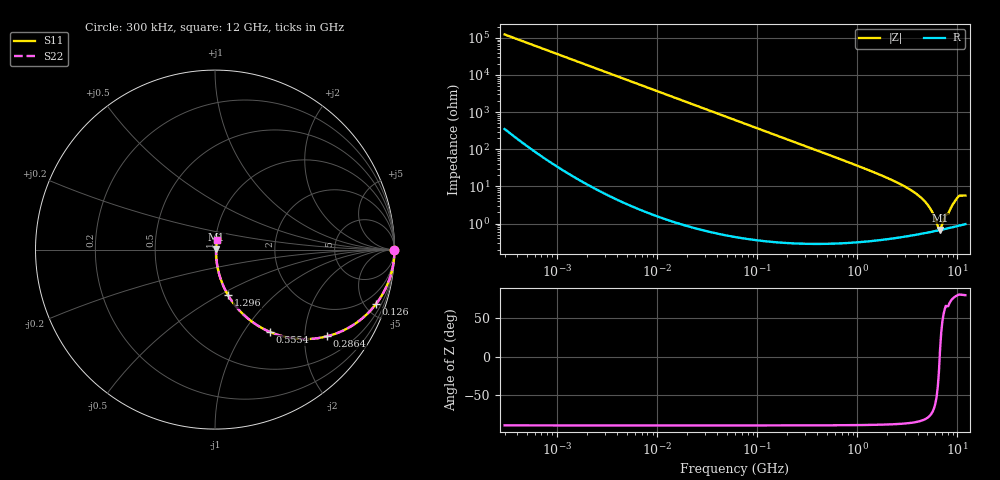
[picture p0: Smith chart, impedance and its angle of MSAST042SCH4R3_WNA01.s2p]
! MSAST042SCH4R3_WNA01  S-PARAMETER MODEL  ( General Type )
! Model Generated by TAIYO YUDEN Corporation (http://www.ty-top.com)
! Version 1.0
! TAIYO YUDEN Control No. 150820
! Copyright(c) 2015 TAIYO YUDEN CO.,LTD. All Rights Reserved.
! Product Description (link to TY-COMPAS)
! https://ds.yuden.co.jp/TYCOMPAS/or/detail?pn=MSAST042SCH4R3BWNA01&u=M
! Products Name : Multilayer Ceramic Capacitors
! Characteristics :
!  Capacitance : 4.3 pF , Rated Voltage : 25V , TCC : CH / C0H
!  Case Size : 0.4 x 0.2 / 0.016 x 0.008 [mm/inch] , Thickness : 0.2 / 0.008 [mm/inch]
!  (Conditions: Temperature = 25 degC , DC Bias Current/Voltage = 0A / 0V)
! External Node Assignments :
!  1  o---| |---o  2
! GND o---------o GND
! Frequency Range : 0.3MHz  -  12000MHz  [ 401 STEP ]
# MHz S RI R 50
! Freq[MHz].  S11 Real  S11 Imag  S21 Real  S21 Imag  S12 Real  S12 Imag  S22 Real  S22 Imag
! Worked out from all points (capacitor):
!   401 points, 300 kHz to 12 GHz, reference 50 ohm
!   read as one part in series: C = 4.31 pF near 316.3 kHz
!   lowest |Z| = 676 mohm at 6.7 GHz (marker M1)
!   series resonance near 6.649 GHz, so ESL is about 130 pH
!   S11 on the Smith chart (normalised r, x): 300 kHz: open; 126 MHz: 1.01, -5.87; 286.4 MHz: 1.01, -2.58; 555.4 MHz: 1.01, -1.32; 1.296 GHz: 1.01, -0.55; 12 GHz: 1.02, +0.11
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0.3  1 -0.000812  2.97e-06 0.000812  2.97e-06 0.000812  1 -0.000812
1.769972  1 -0.00479  2.6e-05 0.00479  2.6e-05 0.00479  1 -0.00479
10.44266  0.9992 -0.0282  0.00081 0.0282  0.00081 0.0282  0.9992 -0.0282
60  0.9742 -0.1581  0.0258 0.1581  0.0258 0.1581  0.9742 -0.1581
125.9782  0.8956 -0.3052  0.1044 0.3052  0.1044 0.3052  0.8956 -0.3052
286.3882  0.6237 -0.4833  0.3763 0.4833  0.3763 0.4833  0.6237 -0.4833
353.9943  0.5201 -0.4982  0.4799 0.4982  0.4799 0.4982  0.5201 -0.4982
555.3718  0.3048 -0.4582  0.6952 0.4582  0.6952 0.4582  0.3048 -0.4582
826.3444  0.1642 -0.367  0.8358 0.367  0.8358 0.367  0.1642 -0.367
1296.429  0.0726 -0.2536  0.9274 0.2536  0.9274 0.2536  0.0726 -0.2536
2088.533  0.0284 -0.1545  0.9716 0.1545  0.9716 0.1545  0.0284 -0.1545
3276.641  0.0118 -0.0842  0.9882 0.0842  0.9882 0.0842  0.0118 -0.0842
4385.161  0.00754 -0.0473  0.9925 0.0473  0.9925 0.0473  0.00754 -0.0473
5278.635  0.00649 -0.0259  0.9935 0.0259  0.9935 0.0259  0.00649 -0.0259
5715.274  0.00636 -0.017  0.9936 0.017  0.9936 0.017  0.00636 -0.017
6354.153  0.00647 -0.00538  0.9935 0.00538  0.9935 0.00538  0.00647 -0.00538
6699.894  0.00664 0.00101  0.9934 -0.00101  0.9934 -0.00101  0.00664 0.00101
6879.757  0.00676 0.00404  0.9932 -0.00404  0.9932 -0.00404  0.00676 0.00404
7448.838  0.00723 0.0129  0.9928 -0.0129  0.9928 -0.0129  0.00723 0.0129
9708.23  0.0102 0.0433  0.9898 -0.0433  0.9898 -0.0433  0.0102 0.0433
10511.28  0.0118 0.0547  0.9882 -0.0547  0.9882 -0.0547  0.0118 0.0547
12000  0.0126 0.0546  0.9874 -0.0546  0.9874 -0.0546  0.0126 0.0546
